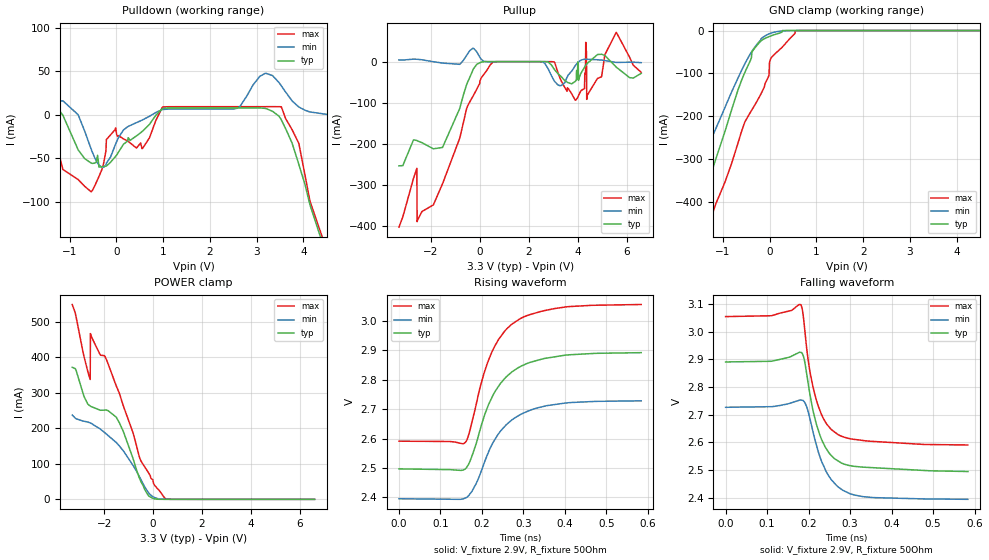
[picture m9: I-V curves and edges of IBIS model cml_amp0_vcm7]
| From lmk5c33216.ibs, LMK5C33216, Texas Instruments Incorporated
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[Model]   cml_amp0_vcm7
Model_type   Output
Polarity   Non-Inverting
Vmeas = 2.7
Vref = 2.9
Cref = 0pF
Rref = 50
|   typ   min   max
C_comp   0.65pF   0.575pF   0.725pF
[Voltage Range]   3.3   3.135   3.465
[Temperature Range]   50   135   -40
[Pullup Reference]   3.3   3.135   3.465
[Pulldown Reference]   0   0   -0
[Power Clamp Reference]   3.3   3.135   3.465
[GND Clamp Reference]   0   0   0
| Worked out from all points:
|   slope of the pulldown table from 0 to 0.495 V, typ, clamps not added: 19.7 ohm
|   falling waveform, V_fixture 2.9V, R_fixture 50Ohm: 20-80 % time 44.9ps typ, 50.3ps min, 42.9ps max; typ from 2.89 V to 2.49 V
|   rising waveform, V_fixture 2.9V, R_fixture 50Ohm: 20-80 % time 76.6ps typ, 80ps min, 72.7ps max; typ from 2.5 V to 2.89 V
[Pulldown]
|   Voltage   I(typ)   I(min)   I(max)
-3.3V     -27.14mA   4.324mA    54.08mA
-2.567V   -19.8mA    3.842mA    100.7mA
-2.558V   -19.24mA   3.8mA      30.12mA
-2.062V   4.942mA    7.968mA    67.27mA
-1.548V   29.06mA    14.36mA    22.78mA
-1.142V   -364.1uA   16.19mA    -62.7mA
-537.9mV  -55.38mA   -39.2mA    -88.39mA
-13.2mV   -47.64mA   -33.49mA   -14.87mA
986.7mV   7.3mA      6.068mA    8.905mA
3.194V    7.34mA     47.71mA    9.467mA
4.679V    -191.6mA   -784.8uA   -183.2mA
6.6V      -291.3mA   5.288mA    -460.8mA
[GND Clamp]
|   Voltage   I(typ)   I(min)   I(max)
-3.3V     -1.161A    -986.5mA   -1.48A
-1.983V   -563.2mA   -494.7mA   -749.9mA
-1.884V   -529.4mA   -456.3mA   -707.9mA
-1.607V   -450.1mA   -352.4mA   -589mA
-1.409V   -387.6mA   -293.5mA   -509.1mA
-1.211V   -320.6mA   -244.1mA   -424.8mA
-537.9mV  -99.97mA   -79.46mA   -216.2mA
-369.6mV  -48.72mA   -47.08mA   -183.7mA
-23.1mV   -14.69mA   -8.348mA   -107.4mA
26.4mV    -12.51mA   -6.259mA   -65.38mA
570.9mV   0A         -9.436uA   -391.3uA
6.6V      0A         0A         0A
[Pullup]
|   Voltage   I(typ)   I(min)   I(max)
-3.3V     -254.1mA   4.269mA    -403.6mA
-2.567V   -192.3mA   5.787mA    -260.3mA
-2.558V   -192.6mA   5.748mA    -390.2mA
-1.894V   -212.6mA   -230.1uA   -349.4mA
541.2mV   -886.4nA   -130.3nA   -969.9uA
3.917V    -47.25mA   -8.81mA    -93.91mA
4.283V    -13.36mA   5.895mA    -65.69mA
4.333V    -8.788mA   5.774mA    47.23mA
4.363V    -6.385mA   5.697mA    23.05mA
4.372V    -5.676mA   5.689mA    -92.02mA
5.58V     -13.45mA   -1.869mA   71.48mA
6.6V      -28.53mA   -2.546mA   -26.23mA
[POWER Clamp]
|   Voltage   I(typ)   I(min)   I(max)
-3.3V     371.7mA    237.1mA    548.5mA
-3.151V   364.4mA    227.2mA    516.2mA
-2.815V   288.8mA    219.8mA    400.7mA
-2.567V   262.8mA    215.2mA    337.4mA
-2.558V   262.4mA    214.9mA    466.8mA
-2.152V   250.9mA    197.5mA    406.7mA
-1.964V   251.4mA    187.3mA    402.2mA
-1.379V   216.1mA    150.7mA    299.1mA
-537.9mV  56.76mA    61.47mA    115.1mA
-191.4mV  10.82mA    19.61mA    75.58mA
481.8mV   75.9uA     118.2uA    3.912mA
6.6V      0A         0A         0A
[Ramp]
R_load = 50
|   typ   min   max
dV/dt_r   0.237102/7.62798e-11   0.19977/7.977e-11   0.278853/7.26025e-11
dV/dt_f   0.237593/4.459e-11   0.199581/4.9922e-11   0.278406/4.29268e-11
[Falling Waveform]
V_fixture = 2.9V
V_fixture_min = 2.735V
V_fixture_max = 3.065V
R_fixture = 50Ohm
C_fixture = 0F
|   Time   V(typ)   V(min)   V(max)
0s        2.89V      2.726V     3.054V
110.2ps   2.893V     2.729V     3.057V
181.1ps   2.925V     2.753V     3.097V
189.2ps   2.902V     2.747V     3.029V
202.2ps   2.782V     2.691V     2.865V
218.9ps   2.664V     2.589V     2.751V
240.1ps   2.583V     2.501V     2.674V
271.3ps   2.532V     2.438V     2.627V
330.9ps   2.51V      2.403V     2.606V
583.8ps   2.494V     2.394V     2.59V
[Rising Waveform]
V_fixture = 2.9V
V_fixture_min = 2.735V
V_fixture_max = 3.065V
R_fixture = 50Ohm
C_fixture = 0F
|   Time   V(typ)   V(min)   V(max)
0s        2.497V     2.395V     2.591V
159.9ps   2.497V     2.398V     2.587V
168.9ps   2.516V     2.408V     2.617V
185.7ps   2.581V     2.446V     2.713V
203.3ps   2.666V     2.509V     2.814V
223.9ps   2.739V     2.578V     2.894V
254.2ps   2.803V     2.64V      2.964V
291.9ps   2.844V     2.681V     3.008V
402.6ps   2.884V     2.721V     3.048V
583.8ps   2.892V     2.728V     3.056V
